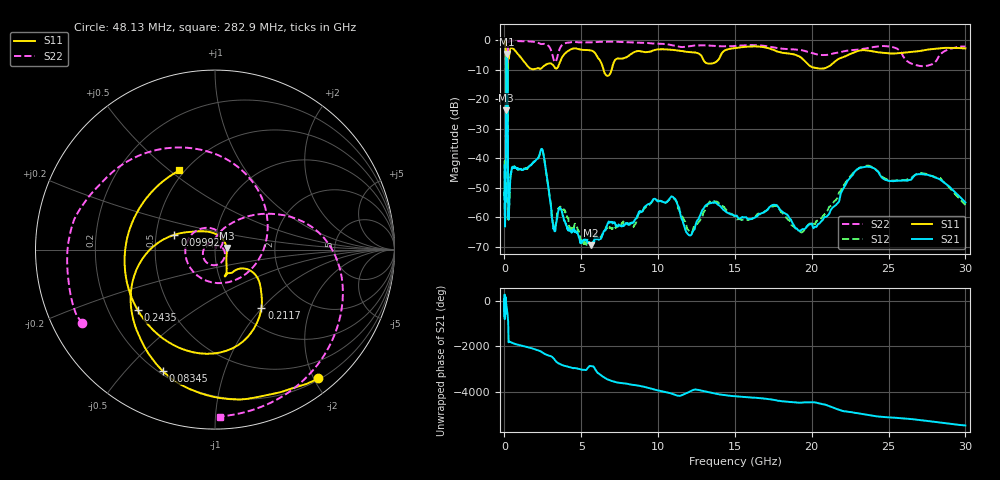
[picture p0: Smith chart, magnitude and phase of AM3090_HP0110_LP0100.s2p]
! Date/Time: Thu, Feb 28, 2019 1:59 PM
! Network Analyzer: Agilent Technologies E8364B Rev: A.07.50.67
! Sweep from 0.010 to 30.000 GHz, 1601 Points, Sweep Type: LOG
! Power Supply: 5.023 V, 0.002 A
# Hz S DB R 50
!freq MagS11 AngS11 MagS21 AngS21 MagS12 AngS12 MagS22 AngS22
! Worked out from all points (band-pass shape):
!   1601 points, 10 MHz to 30 GHz, reference 50 ohm
!   highest |S21| = -4.73 dB at 149.9 MHz (marker M1); lowest = -69.3 dB at 5.64 GHz (marker M2)
!   |S21| within 3 dB of the highest: 110 MHz to 197.5 MHz (87.54 MHz wide, 56.9 % of centre)
!   lowest |S11| = -23.7 dB at 107.7 MHz (marker M3), VSWR 1.14, Z = 56.9 + j1.01 ohm
!   |S11| at or under -10 dB: 98.5 MHz to 200.8 MHz (102.3 MHz wide, 68.4 % of centre); 6.447 GHz to 6.978 GHz (531.2 MHz wide, 7.91 % of centre)
!   |S22| runs from -40.0 to -0.1 dB; largest |S21 - S12| = 0.013
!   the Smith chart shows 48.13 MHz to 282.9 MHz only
!   S11 on the Smith chart (normalised r, x): 48.13 MHz: 0.22, -2.06; 83.45 MHz: 0.22, -0.64; 99.92 MHz: 0.62, +0.11; 211.7 MHz: 1.26, -0.99; 243.5 MHz: 0.32, -0.31; 282.9 MHz: 0.47, +0.54
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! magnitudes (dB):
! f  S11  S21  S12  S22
! 10 MHz  -0.2  -42.5  -41.0  -0.5
! 38.04 MHz  -0.5  -60.9  -61.0  -1.3
! 48.13 MHz  -0.7  -49.9  -49.9  -1.5
! 83.45 MHz  -2.7  -49.6  -49.7  -5.5
! 99.92 MHz  -12.4  -16.0  -15.9  -15.0
! 107.7 MHz  -23.7  -8.6  -8.6  -16.4
! 132.2 MHz  -16.1  -5.0  -5.0  -39.8
! 144.7 MHz  -16.5  -4.8  -4.7  -27.9
! 149.9 MHz  -16.4  -4.7  -4.7  -24.6
! 186.8 MHz  -14.2  -6.1  -6.1  -26.2
! 211.7 MHz  -7.6  -15.0  -14.9  -10.3
! 243.5 MHz  -5.2  -57.7  -56.9  -1.4
! 282.9 MHz  -6.3  -59.2  -56.2  -0.6
! 550.5 MHz  -2.9  -43.2  -42.9  -0.2
! 2.084 GHz  -9.7  -40.4  -40.5  -0.8
! 2.507 GHz  -9.0  -37.8  -38.0  -1.3
! 3.204 GHz  -8.7  -63.7  -63.4  -6.7
! 5.64 GHz  -3.5  -69.3  -66.3  -0.8
! 7.926 GHz  -5.9  -62.1  -62.1  -0.7
! 19.51 GHz  -6.9  -64.1  -64.4  -3.6
! 23.48 GHz  -3.4  -42.9  -42.6  -2.9
! 30 GHz  -2.8  -55.0  -55.8  -2.2
